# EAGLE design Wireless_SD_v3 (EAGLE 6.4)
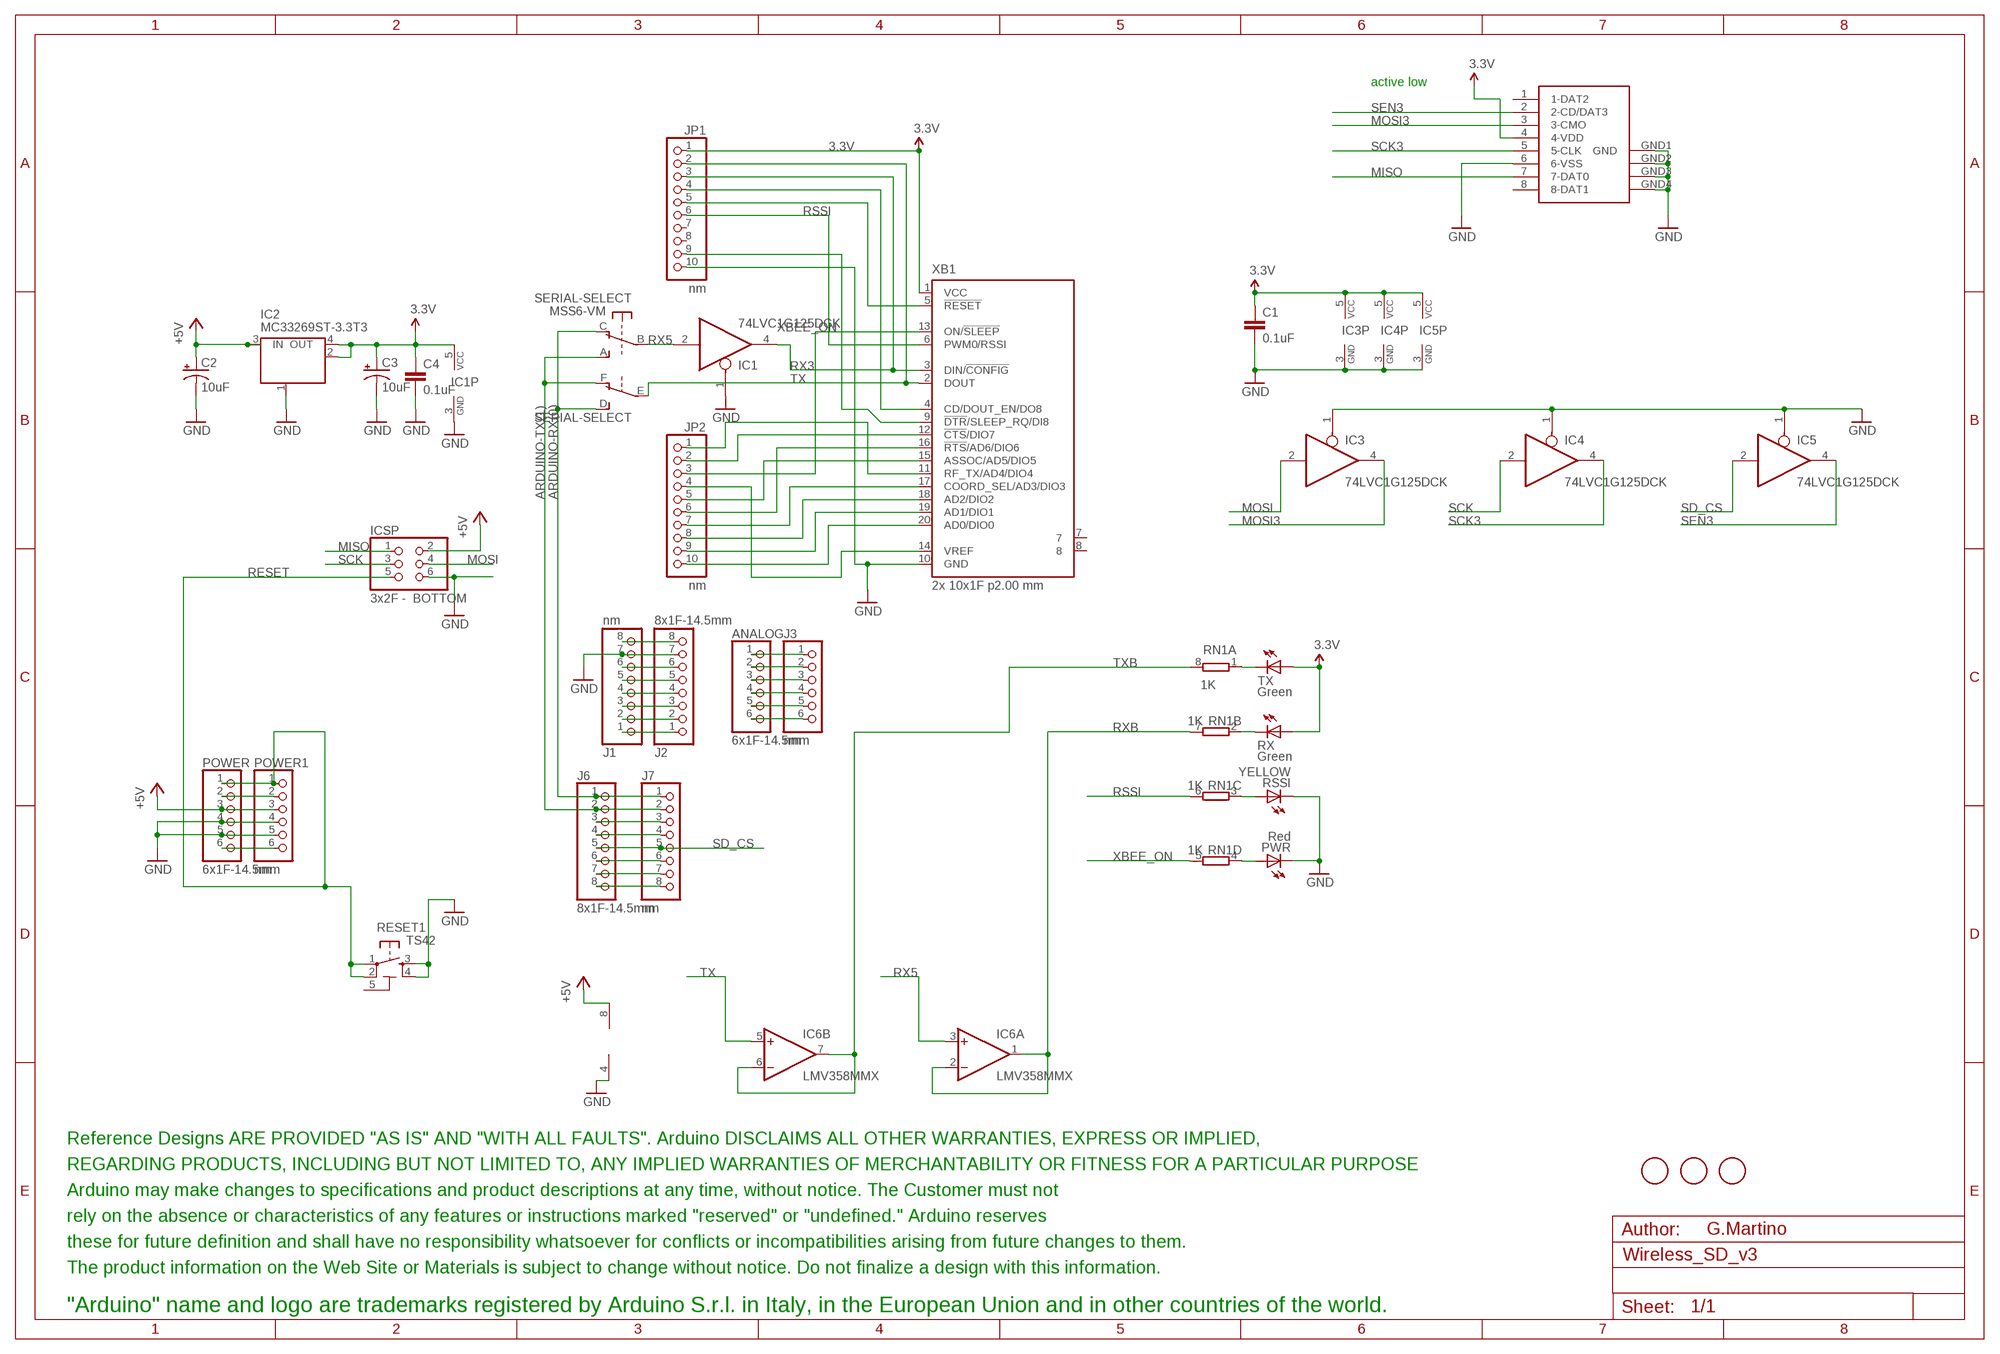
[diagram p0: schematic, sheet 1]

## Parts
A1  FIDUCIALMOUNT  [FIDUCIA-MOUNT]
A2  FIDUCIALMOUNT  [FIDUCIA-MOUNT]
A3  FIDUCIALMOUNT  [FIDUCIA-MOUNT]
ANALOG  6x1F-14.5mm  PINHD-1X6  [1X06]
C1  0.1uF  CAP0603-CAP  [0603-CAP]
C2  10uF  CAP_POL1206  [EIA3216]
C3  10uF  CAP_POL1206  [EIA3216]
C4  0.1uF  CAP0603-CAP  [0603-CAP]
IC1  74LVC1G125DCK  [SC70-5]
IC2  MC33269ST-3.3T3  [SOT223]
IC3  74LVC1G125DCK  [SC70-5]
IC4  74LVC1G125DCK  [SC70-5]
IC5  74LVC1G125DCK  [SC70-5]
IC6  LMV358MMX  [MSOP08]
ICSP  3x2F - BOTTOM  PINHD-2X3  [2X03]
J1  nm  PINHD-1X8  [1X08]
J2  8x1F-14.5mm  PINHD-1X8  [1X08]
J3  nm  PINHD-1X6  [1X06]
J6  8x1F-14.5mm  PINHD-1X8  [1X08]
J7  nm  PINHD-1X8  [1X08]
JP1  nm  PINHD-1X10  [1X10]
JP2  nm  PINHD-1X10  [1X10]
POWER  6x1F-14.5mm  PINHD-1X6  [1X06]
POWER1  nm  PINHD-1X6  [1X06]
PWR  Red  LEDCHIP-LED0805  [CHIP-LED0805]
RESET1  TS42  [TS42]
RN1  1K  4R-NCAY16  [CAY16]
RSSI  YELLOW  LEDCHIP-LED0805  [CHIP-LED0805]
RX  Green  LEDCHIP-LED0805  [CHIP-LED0805]
SERIAL-SELECT  MSS6-VM  [MSS6-V]
TX  Green  LEDCHIP-LED0805  [CHIP-LED0805]
U$2  DISCLAIMER-SMALL  [DISCLAIMER]
X1  SDCARD-15TW-8821  [SDCARD-15TW-8821]
XB1  2x 10x1F p2.00 mm  XBEE-PRO  [XBEE-PRO]

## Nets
3.3V: C1.1 C3.A(+) C4.1 IC1.5(VCC) IC2.2(OUT) IC2.4(OUT) IC3.5(VCC) IC4.5(VCC) IC5.5(VCC) JP1.1 RX.A TX.A X1.4(4-VDD) XB1.1(VCC)
+5V: C2.A(+) IC2.3(IN) IC6.8(P:V+) ICSP.2 POWER1.3 POWER.3
ARDUINO-RX(0): J6.1 J7.1 SERIAL-SELECT.C(O) SERIAL-SELECT.D(S)
ARDUINO-TX(1): J6.2 J7.2 SERIAL-SELECT.A(S) SERIAL-SELECT.F(O)
GND: C1.2 C2.C(-) C3.C(-) C4.2 IC1.1(OE) IC1.3(GND) IC2.1(GND/ADJ) IC3.1(OE) IC3.3(GND) IC4.1(OE) IC4.3(GND) IC5.1(OE) IC5.3(GND) IC6.4(P:V-) ICSP.6 J1.7 J2.7 JP1.10 POWER1.4 POWER1.5 POWER.4 POWER.5 PWR.C RESET1.3 RESET1.4 RSSI.C X1.6(6-VSS) X1.GND1(GND) X1.GND2(GND1) X1.GND3(GND2) X1.GND4(GND3) XB1.10(GND)
MISO: ICSP.1 X1.7(7-DAT0)
MOSI: IC3.2(I) ICSP.4
MOSI3: IC3.4(O) X1.3(3-CMO)
N$1: RN1.1 TX.C
N$2: J1.1 J2.1
N$5: RN1.2 RX.C
N$6: J1.2 J2.2
N$7: J1.3 J2.3
N$9: J1.6 J2.6
N$10: J6.3 J7.3
N$11: J6.4 J7.4
N$13: J6.6 J7.6
N$14: J6.7 J7.7
N$15: J6.8 J7.8
N$16: RN1.3 RSSI.A
N$18: ANALOG.1 J3.1
N$19: ANALOG.2 J3.2
N$20: ANALOG.3 J3.3
N$21: ANALOG.4 J3.4
N$22: ANALOG.5 J3.5
N$23: ANALOG.6 J3.6
N$24: JP2.10 XB1.20(AD0/DIO0)
N$25: JP2.9 XB1.19(AD1/DIO1)
N$27: J1.5 J2.5
N$28: JP2.8 XB1.18(AD2/DIO2)
N$29: PWR.A RN1.4
N$30: POWER1.6 POWER.6
N$33: JP2.7 XB1.17(COORD_SEL/AD3/DIO3)
N$34: JP2.6 XB1.16(!RTS!/AD6/DIO6)
N$36: JP2.5 XB1.15(ASSOC/AD5/DIO5)
N$37: JP2.4 XB1.14(VREF)
N$39: JP2.2 XB1.12(!CTS!/DIO7)
N$41: JP2.1 XB1.11(RF_TX/AD4/DIO4)
N$43: JP1.4 XB1.4(CD/DOUT_EN/DO8)
N$48: JP1.5 XB1.5(!RESET)
N$50: JP1.9 XB1.9(!DTR!/SLEEP_RQ/DI8)
N$61: J1.4 J2.4
N$222: J1.8 J2.8
N$223: POWER1.2 POWER.2
RESET: ICSP.5 POWER1.1 POWER.1 RESET1.1 RESET1.2
RSSI: JP1.6 RN1.6 XB1.6(PWM0/RSSI)
RX3: IC1.4(O) JP1.3 XB1.3(DIN/!CONFIG)
RX5: IC1.2(I) IC6.3(A:+IN) SERIAL-SELECT.B(P)
RXB: IC6.1(A:OUT) IC6.2(A:-IN) RN1.7
SCK: IC4.2(I) ICSP.3
SCK3: IC4.4(O) X1.5(5-CLK)
SD_CS: IC5.2(I) J6.5 J7.5
SEN3: IC5.4(O) X1.2(2-CD/DAT3)
TX: IC6.5(B:+IN) JP1.2 SERIAL-SELECT.E(P) XB1.2(DOUT)
TXB: IC6.6(B:-IN) IC6.7(B:OUT) RN1.8
XBEE_ON: JP2.3 RN1.5 XB1.13(ON/!SLEEP)
Unconnected: JP1.7 JP1.8 X1.1(1-DAT2) X1.8(8-DAT1) XB1.7 XB1.8

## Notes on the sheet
- active low
- G.Martino

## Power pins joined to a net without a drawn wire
5-GND: RESET1.5(5-GND)

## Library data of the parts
A1-A3 = Smartprj:FIDUCIALMOUNT
ANALOG J3 POWER POWER1 = pinhead:PINHD-1X6: PIN HEADER
C1 C4 = SparkFun:CAP: Capacitor
C2 C3 = SparkFun:CAP_POL: Capacitor Polarized
IC1 IC3-IC5 = 74xx-little-us:74*1G125: Single Bus Buffer Gate with 3-State Output
IC2 = linear:MC33269ST*: Adjustable Output Low Dropout Voltage Regulator 800 mA Source: http://www.onsemi.com/pub/Collateral/MC33269-D.PDF
IC6 = linear:LMV358?*: Dual General Purpose, Low Voltage, Rail-to-Rail Output Operational Amplifiers Source: http://www.national.com/mpf/LM/LMV321.html http://www.national.com/dt/lmv_qual.pdf
ICSP = pinhead:PINHD-2X3: PIN HEADER
J1 J2 J6 J7 = pinhead:PINHD-1X8: PIN HEADER
JP1 JP2 = pinhead:PINHD-1X10: PIN HEADER
PWR RSSI RX TX = led:LED: LED
RESET1 = st-mod v1.4:TS42: TS42 Dongnan Electronics Tact switch VDC 12V - 50mA
RN1 = resistor-dil:4R-N: Array Chip Resistor Source: RS Component / Phycomp
SERIAL-SELECT = Smartprj:MSS6-V
U$2 = Misc:DISCLAIMER-SMALL: DISCLAIMER
X1 = st-mod v1.3:SDCARD-15TW-8821: SD Card SDCARD 15TW 8821
XB1 = maxstream:XBEE: XBee (TM) /XBee-PRO(TM) OEM RF Modules Source: MaxStream, Inc. xbee_productmanual.pdf

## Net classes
0 default: width 0.203 mm, drill 0.559 mm, clearance 0.203 mm
1 power: width 0.152 mm, drill 0.61 mm, clearance 0.152 mm
2 gnd: width 0.203 mm, drill 0.559 mm, clearance 0.203 mm

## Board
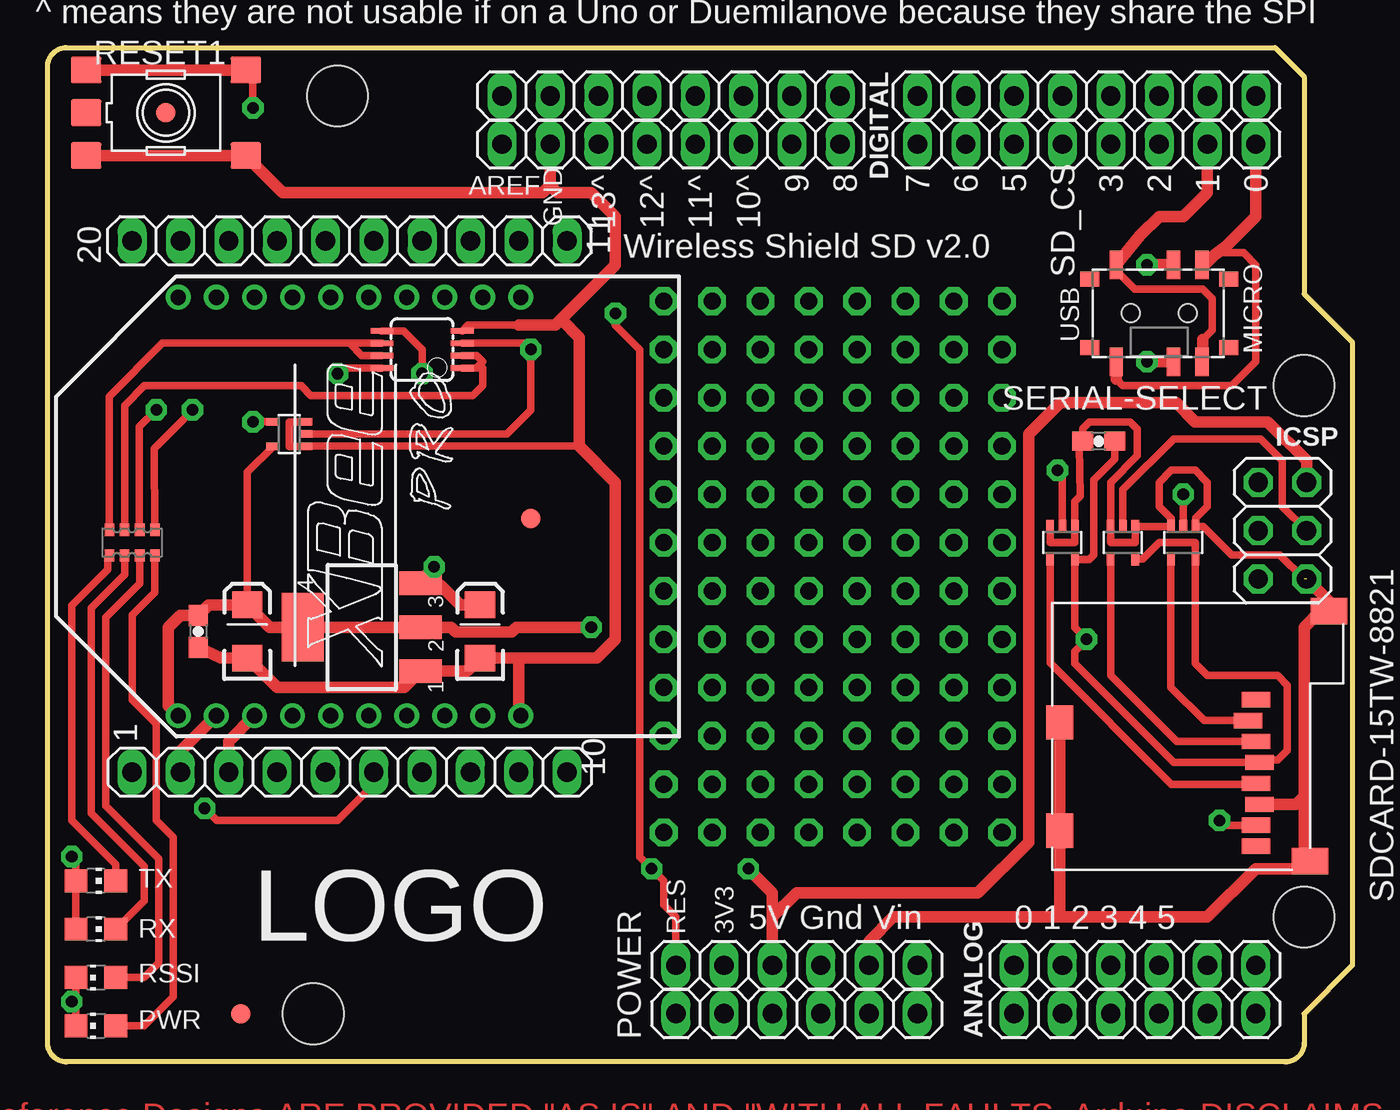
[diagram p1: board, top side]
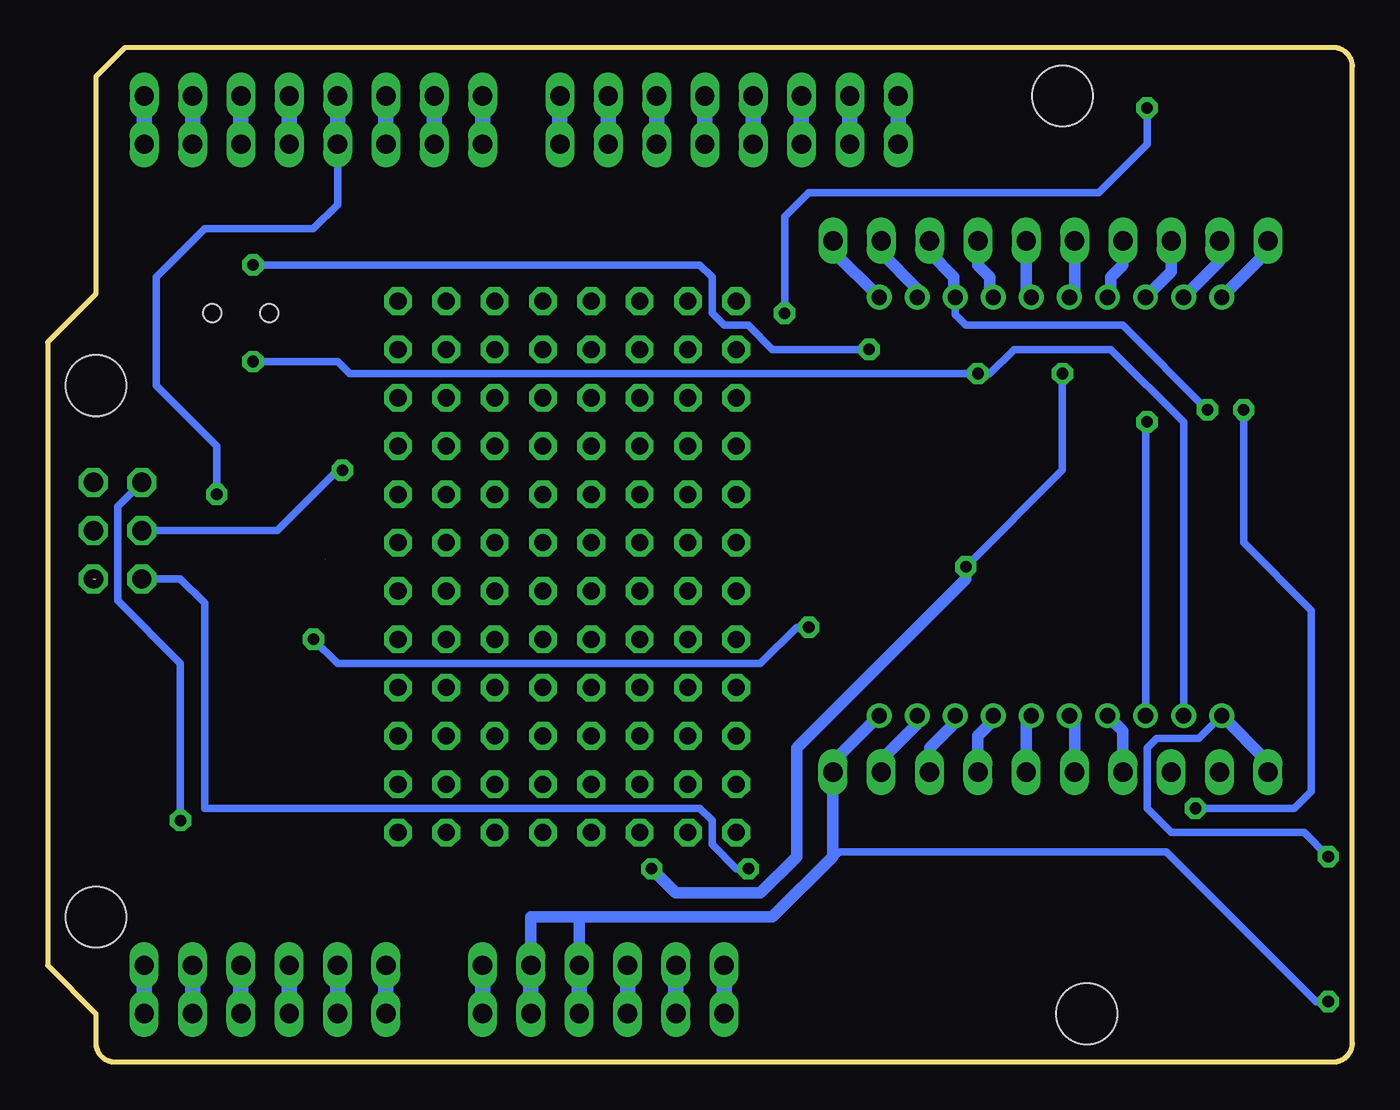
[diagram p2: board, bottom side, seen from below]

Size 68.58 x 53.34 mm. Coordinates in mm from the lower left corner, seen from the top.
Outline: 64.52,53.34 66.04,51.82 66.04,40.39 68.58,37.85 68.58,5.08 66.04,2.54 66.04,1 arc-90 65.04,0 1,0 arc-90 0,1 0,52.34 arc-90 1,53.34 64.52,53.34
Copper layers (1*16): Top 0.035mm / dielectric 1.5mm / Bottom 0.035mm
Design rules "ArduinoUno *": minimum track width 12mil, minimum drill 32mil, track to track 12mil, track to pad 12mil, pad to pad 12mil, via to via 12mil, smd to smd 12mil, copper to edge 32mil, drill to drill 16mil, minimum pad ring 10mil, minimum via ring 10mil, stop-mask expansion 2mil, vias tented up to drill 30mil, thermal gap 10mil
Holes 3.2 mm at 15.24,50.8 66.04,7.62 66.04,35.56 13.97,2.54

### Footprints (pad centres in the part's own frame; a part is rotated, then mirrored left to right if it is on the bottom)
FIDUCIA-MOUNT = smd 1.016 x 1.016: P$1 0,0
1X06 = drill 1.016 long: 1 -6.35,0; 2 -3.81,0; 3 -1.27,0; 4 1.27,0; 5 3.81,0; 6 6.35,0
0603-CAP = smd 1.1 x 1: 1 -0.85,0; 2 0.85,0
EIA3216 = smd 1.4 x 1.6: A 1.4,0; C -1.4,0
SC70-5 = smd 0.4 x 0.7: 1 -0.65,-0.85; 2 0,-0.85; 3 0.65,-0.85; 4 0.65,0.85; 5 -0.65,0.85
SOT223 = smd 1.219 x 2.235: 1 -2.311,-3.099; 2 0,-3.099; 3 2.311,-3.099 | smd 3.6 x 2.2: 4 0,3.099
MSOP08 = smd 0.3 x 1.2: 1 -0.976,-2.113; 2 -0.326,-2.113; 3 0.324,-2.113; 4 0.974,-2.113; 5 0.974,2.112; 6 0.324,2.112; 7 -0.326,2.112; 8 -0.976,2.112
2X03 = drill 1.016 octagon: 1 -2.54,-1.27; 2 -2.54,1.27; 3 0,-1.27; 4 0,1.27; 5 2.54,-1.27; 6 2.54,1.27
1X08 = drill 1.016 long: 1 -8.89,0; 2 -6.35,0; 3 -3.81,0; 4 -1.27,0; 5 1.27,0; 6 3.81,0; 7 6.35,0; 8 8.89,0
1X10 = drill 1.016 long: 1 -11.43,0; 2 -8.89,0; 3 -6.35,0; 4 -3.81,0; 5 -1.27,0; 6 1.27,0; 7 3.81,0; 8 6.35,0; 9 8.89,0; 10 11.43,0
CHIP-LED0805 = smd 1.2 x 1.2: A 0,-1.05; C 0,1.05
TS42 = smd 1.6 x 1.4: 1 -4.2,2.25; 2 4.2,2.25; 3 -4.2,-2.25; 4 4.2,-2.25; 5 -4.2,0
CAY16 = smd 0.5 x 0.65: 1 -1.2,-0.675; 2 -0.4,-0.675; 3 0.4,-0.675; 4 1.2,-0.675; 5 1.2,0.675; 6 0.4,0.675; 7 -0.4,0.675; 8 -1.2,0.675
MSS6-V = smd 1 x 0.8: 7 -3.65,1.8; 8 -3.65,-1.8; 9 3.65,1.8; 10 3.65,-1.8 | smd 0.7 x 1.5: A -2.25,2.55; B 0.75,2.55; C 2.25,2.55; D -2.25,-2.55; E 0.75,-2.55; F 2.25,-2.55 | hole 0.95: -1.5,0; 1.5,0
SDCARD-15TW-8821 = smd 0.8 x 1.5: 1 0,0; 2 1.1,-0.4; 3 2.2,0; 4 3.3,0.2; 5 4.4,0; 6 5.5,0.2; 7 6.6,0; 8 7.7,0 | smd 1.4 x 1.9: GND1 -4.66,3.85; GND2 8.49,2.85 | smd 1.8 x 1.4: GND3 1.19,-10.3; GND4 6.89,-10.3
XBEE-PRO = drill 0.8 pad 1.27: 1 -11,9; 2 -11,7; 3 -11,5; 4 -11,3; 5 -11,1; 6 -11,-1; 7 -11,-3; 8 -11,-5; 9 -11,-7; 10 -11,-9; 11 11,-9; 12 11,-7; 13 11,-5; 14 11,-3; 15 11,-1; 16 11,1; 17 11,3; 18 11,5; 19 11,7; 20 11,9

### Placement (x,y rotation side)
A1  10.16,2.54 0 top
A2  6.22,49.91 0 top
A3  25.4,28.57 0 top
ANALOG  57.15,2.54 0 top
C1  55.24,32.64 180 top
C2  22.73,22.64 90 top
C3  10.49,22.64 90 top
C4  7.92,22.64 270 top
IC1  12.7,33.02 90 top
IC2  16.51,22.86 90 top
IC3  56.52,27.3 180 top
IC4  53.34,27.3 180 top
IC5  59.69,27.3 180 top
IC6  19.68,37.47 90 top
ICSP  64.9,27.94 270 top
J1  32.77,48.26 180 top
J2  32.77,50.8 180 top
J3  57.15,5.08 0 top
J6  54.61,50.8 180 top
J7  54.61,48.26 180 top
JP1  15.88,15.24 0 top
JP2  15.88,43.18 180 top
POWER  39.37,2.54 0 top
POWER1  39.37,5.08 0 top
PWR  2.54,1.91 90 top
RESET1  6.22,49.91 0 top
RN1  4.45,27.3 0 top
RSSI  2.54,4.45 90 top
RX  2.54,6.99 270 top
SERIAL-SELECT  58.42,39.37 0 top
TX  2.54,9.53 270 top
U$2  not placed on the board
X1  63.5,19.05 270 top
XB1  15.88,29.21 90 top

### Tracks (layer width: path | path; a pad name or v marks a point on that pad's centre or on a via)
3.3V  (via drill 0.61)  (1 unrouted)
  Top 0.406: C1.1 56.09,31.71 54.99,30.61 54.99,26.67 54.74,26.42 54.03,26.42 IC4.5 | C3.A 10.49,31.02 IC1.5 | 60.33,26.47 60.33,20.95 60.96,20.32 64.64,20.32 65.15,19.81 65.15,16.38 64.64,15.88 63.83,15.88 X1.4 59.18,15.75 53.98,20.95 53.98,21.59 v54.61,22.23 53.98,22.86 53.98,26.44 | RX.A TX.A 1.49,10.57 v1.27,10.79 | IC3.5 57.57,26.45 58.42,27.3 60.33,27.3 60.33,26.47 | 60.33,26.47 IC5.5
  Top 0.61: v28.57,22.86 24.64,22.86 24.38,22.61 21.46,22.61 21.21,22.86 IC2.2 IC2.4 11.67,22.86 C3.A 8.46,24.04 C4.1 6.97,23.48 6.35,22.86 6.35,18.72 6.37,18.72 XB1.1
  Bottom 0.406: v1.27,10.79 2.54,12.06 9.53,12.06 10.79,13.34 10.79,16.51 10.29,17.02 8.07,17.02 XB1.1 | v28.57,22.86 29.21,22.86 31.11,20.95 53.34,20.95 v54.61,22.23
  Bottom 0.61: JP1.1 4.45,15.78 XB1.1
+5V  (via drill 0.61)
  Top 0.406: IC6.8 15.53,36.49 v15.24,36.2
  Top 0.61: 38.1,7.62 POWER1.3 | 38.1,7.62 39.37,8.89 48.9,8.89 51.56,11.56 51.56,33.02 53.21,34.67 59.31,34.67 60.33,33.66 64.14,33.66 66.17,31.62 ICSP.2 | 38.1,7.62 38.1,8.89 v36.83,10.16 | v20.32,26.04 19.61,25.32 IC2.3 19.7,25.08 20.64,25.08 21.68,24.04 C2.A
  Bottom 0.406: v15.24,36.2 15.24,31.11 v20.32,26.04
  Bottom 0.61: v36.83,10.16 35.56,8.89 31.11,8.89 29.21,10.79 29.21,16.51 20.32,25.4 v20.32,26.04
  Bottom 0.813: POWER1.3 POWER.3
ARDUINO-RX(0)
  Top 0.406: SERIAL-SELECT.C 60.97,41.92 61.59,42.55 62.87,42.55 63.5,41.91 63.5,36.83 62.23,35.56 56.52,35.56 56.17,35.91
  Top 0.61: SERIAL-SELECT.C 61.94,42.89 63.5,44.45 J7.1 | SERIAL-SELECT.D 56.17,35.91
  Bottom 0.813: J7.1 J6.1
ARDUINO-TX(1)
  Top 0.406: SERIAL-SELECT.A 56.17,41.62 57.15,40.64 60.71,40.64 61.21,40.13 61.21,38.48 60.71,37.97 | SERIAL-SELECT.F 60.71,36.86
  Top 0.61: SERIAL-SELECT.A 57.44,43.47 58.42,44.45 59.69,44.45 60.96,45.72 J7.2 | 60.71,36.86 60.71,37.97
  Bottom 0.813: J7.2 J6.2
GND  (via drill 0.61)  (1 unrouted)
  Top 0.406: PWR.C RSSI.C 1.49,3.4 v1.27,3.17 | 66.04,25.4 64.77,26.67 62.23,26.67 60.74,28.16 IC5.1 60.34,28.59 60.96,29.21 60.96,30.48 60.33,31.11 59.05,31.11 58.42,30.48 58.42,29.21 59.05,28.57 59.05,28.17 IC5.3 IC3.1 57.16,27.32 57.15,27.3 55.88,27.3 55.88,28.14 IC3.3 55.87,30.46 57.28,31.88 57.28,33.27 56.9,33.66 54.74,33.66 54.4,33.31 C1.2 54.23,32.47 54.23,32.38 54.27,29.76 53.99,29.48 IC4.1 53.98,28.14 53.98,27.3 52.7,27.3 52.69,27.32 IC4.3 | 24.77,38.73 22.09,38.73 IC6.4 | IC1.3 13.54,33.66 12.7,33.66 12.7,32.38 12.71,32.37 IC1.1 13.56,32.38 27.94,32.38
  Top 0.61: RESET1.3 RESET1.4 12.36,45.72 26.04,45.72 26.42,46.1 | C4.2 9.1,21.23 C3.C 10.52,21.23 12.06,19.68 18.75,19.68 IC2.1 22.05,20.55 C2.C 24.77,21.23 | XB1.10 24.77,18.32 24.77,21.23 | 26.42,46.1 J1.7 | 24.77,38.73 26.67,38.73 26.99,39.05 | 26.99,39.05 29.84,41.91 29.84,44.45 28.57,45.72 26.8,45.72 26.42,46.1 | 26.99,39.05 27.94,38.1 27.94,32.38 29.84,30.48 29.84,22.23 28.86,21.23 24.77,21.23 | POWER1.5 43.18,6.35 44.45,7.62 53.34,7.62 | 53.34,7.62 60.96,7.62 63.5,10.16 65.95,10.16 X1.GND2 66.04,10.87 66.04,13.97 | 66.04,13.97 66.04,22.86 66.89,23.71 X1.GND1 67.35,24.22 ICSP.6 | X1.6 65.62,13.55 66.04,13.97 | X1.GND4 X1.GND3 | X1.GND4 53.2,11.57 53.34,11.43 53.34,12.02 X1.GND4 | X1.GND4 53.2,7.76 53.34,7.62
  Bottom 0.406: v1.27,3.17 1.91,3.17 9.78,11.05 26.92,11.05 27.3,10.79
  Bottom 0.61: XB1.10 27.3,15.78 JP1.10 27.3,10.79 30.48,7.62 40.64,7.62 | 40.64,7.62 POWER1.4 | POWER1.5 43.18,7.62 40.64,7.62
  Bottom 0.813: J1.7 J2.7 | POWER1.4 POWER.4 | POWER1.5 POWER.5
MISO  (via drill 0.61)
  Top 0.406: X1.7 61.84,12.45 v61.59,12.7
  Bottom 0.406: v61.59,12.7 61.59,20.95 64.9,24.26 64.9,29.21 ICSP.1
MOSI
  Top 0.406: ICSP.4 64.9,29.21 64.9,31.62 63.75,32.77 59.18,32.77 56.52,30.1 IC3.2
MOSI3
  Top 0.406: IC3.4 55.87,20.34 59.35,16.85 X1.3
N$1
  Top 0.406: TX.C 3.59,10.38 1.27,12.7 1.27,24 3.17,25.91 3.17,26.56 RN1.1
N$2
  Bottom 0.813: J1.1 J2.1
N$5
  Top 0.406: RN1.2 4.04,25.64 2.29,23.88 2.29,13.08 5.08,10.29 5.08,8.47 RX.C
N$6
  Bottom 0.813: J1.2 J2.2
N$7
  Bottom 0.813: J1.3 J2.3
N$8  (via drill 0.9 pad 1.45)
  other vias: 34.92,32.38
N$9
  Bottom 0.813: J1.6 J2.6
N$10
  Bottom 0.813: J7.3 J6.3
N$11
  Bottom 0.813: J7.4 J6.4
N$13
  Bottom 0.813: J7.6 J6.6
N$14
  Bottom 0.813: J7.7 J6.7
N$15
  Bottom 0.813: J7.8 J6.8
N$16
  Top 0.406: RSSI.A 5.08,4.45 5.84,5.21 5.84,10.67 3.05,13.46 3.05,23.37 4.84,25.16 RN1.3
N$18
  Bottom 0.813: ANALOG.1 J3.1
N$19
  Bottom 0.813: ANALOG.2 J3.2
N$20
  Bottom 0.813: ANALOG.3 J3.3
N$21
  Bottom 0.813: ANALOG.4 J3.4
N$22
  Bottom 0.813: ANALOG.5 J3.5
N$23
  Bottom 0.813: ANALOG.6 J3.6
N$24
  Bottom 0.61: JP2.10 4.45,42.64 XB1.20
N$25
  Bottom 0.61: JP2.9 6.99,42.1 XB1.19
N$27
  Bottom 0.813: J1.5 J2.5
N$28
  Bottom 0.61: JP2.8 9.53,41.56 XB1.18
N$29
  Top 0.406: PWR.A 5.08,1.91 6.6,3.43 6.6,11.81 5.71,12.7 5.71,17.78 4.45,19.05 4.45,23.5 5.64,24.7 RN1.4
N$30
  Bottom 0.813: POWER.6 POWER1.6
N$32  (via drill 0.9 pad 1.45)
  other vias: 34.92,40.01
N$33
  Bottom 0.61: JP2.7 12.06,41.91 12.7,41.27 12.7,40.38 XB1.17
N$34
  Bottom 0.61: JP2.6 14.61,40.48 XB1.16
N$35  (via drill 0.9 pad 1.45)
  other vias: 34.92,37.47
N$36
  Bottom 0.61: JP2.5 17.14,40.48 XB1.15
N$37
  Bottom 0.61: JP2.4 19.68,41.91 19.05,41.27 19.05,40.38 XB1.14
N$38  (via drill 0.9 pad 1.45)
  other vias: 34.92,34.92
N$39
  Bottom 0.61: JP2.2 24.77,42.55 22.86,40.64 22.86,40.23 XB1.12
N$41
  Bottom 0.61: JP2.1 27.3,42.64 XB1.11
N$43
  Bottom 0.61: JP1.4 12.06,17.4 XB1.4
N$48
  Bottom 0.61: JP1.5 14.61,17.94 XB1.5
N$50
  Bottom 0.61: JP1.9 24.77,15.88 22.86,17.78 22.86,18.2 XB1.9
N$55  (via drill 0.9 pad 1.45)
  other vias: 34.92,29.84
N$57  (via drill 0.9 pad 1.45)
  other vias: 34.92,27.3
N$58  (via drill 0.9 pad 1.45)
  other vias: 34.92,24.77
N$60  (via drill 0.9 pad 1.45)
  other vias: 50.16,40.01
N$61
  Bottom 0.813: J1.4 J2.4
N$62  (via drill 0.9 pad 1.45)
  other vias: 45.09,40.01
N$63  (via drill 0.9 pad 1.45)
  other vias: 34.92,22.23
N$64  (via drill 0.9 pad 1.45)
  other vias: 40.01,40.01
N$65  (via drill 0.9 pad 1.45)
  other vias: 34.92,19.68
N$66  (via drill 0.9 pad 1.45)
  other vias: 34.92,17.14
N$67  (via drill 0.9 pad 1.45)
  other vias: 34.92,14.61
N$68  (via drill 0.9 pad 1.45)
  other vias: 34.92,12.06
N$69  (via drill 0.9 pad 1.45)
  other vias: 32.38,32.38
N$70  (via drill 0.9 pad 1.45)
  other vias: 32.38,29.84
N$71  (via drill 0.9 pad 1.45)
  other vias: 32.38,27.3
N$72  (via drill 0.9 pad 1.45)
  other vias: 32.38,24.77
N$75  (via drill 0.9 pad 1.45)
  other vias: 32.38,22.23
N$76  (via drill 0.9 pad 1.45)
  other vias: 42.55,40.01
N$77  (via drill 0.9 pad 1.45)
  other vias: 37.47,40.01
N$79  (via drill 0.9 pad 1.45)
  other vias: 50.16,37.47
N$80  (via drill 0.9 pad 1.45)
  other vias: 45.09,37.47
N$81  (via drill 0.9 pad 1.45)
  other vias: 40.01,37.47
N$82  (via drill 0.9 pad 1.45)
  other vias: 32.38,19.68
N$85  (via drill 0.9 pad 1.45)
  other vias: 47.62,40.01
N$86  (via drill 0.9 pad 1.45)
  other vias: 42.55,37.47
N$87  (via drill 0.9 pad 1.45)
  other vias: 37.47,37.47
N$89  (via drill 0.9 pad 1.45)
  other vias: 50.16,34.92
N$90  (via drill 0.9 pad 1.45)
  other vias: 45.09,34.92
N$91  (via drill 0.9 pad 1.45)
  other vias: 40.01,34.92
N$92  (via drill 0.9 pad 1.45)
  other vias: 32.38,17.14
N$95  (via drill 0.9 pad 1.45)
  other vias: 47.62,34.92
N$96  (via drill 0.9 pad 1.45)
  other vias: 42.55,34.92
N$97  (via drill 0.9 pad 1.45)
  other vias: 37.47,34.92
N$99  (via drill 0.9 pad 1.45)
  other vias: 50.16,32.38
N$100  (via drill 0.9 pad 1.45)
  other vias: 45.09,32.38
N$101  (via drill 0.9 pad 1.45)
  other vias: 40.01,32.38
N$102  (via drill 0.9 pad 1.45)
  other vias: 32.38,14.61
N$105  (via drill 0.9 pad 1.45)
  other vias: 47.62,32.38
N$106  (via drill 0.9 pad 1.45)
  other vias: 42.55,32.38
N$107  (via drill 0.9 pad 1.45)
  other vias: 37.47,32.38
N$109  (via drill 0.9 pad 1.45)
  other vias: 50.16,29.84
N$110  (via drill 0.9 pad 1.45)
  other vias: 45.09,29.84
N$111  (via drill 0.9 pad 1.45)
  other vias: 40.01,29.84
N$112  (via drill 0.9 pad 1.45)
  other vias: 32.38,12.06
N$115  (via drill 0.9 pad 1.45)
  other vias: 47.62,29.84
N$116  (via drill 0.9 pad 1.45)
  other vias: 42.55,29.84
N$117  (via drill 0.9 pad 1.45)
  other vias: 37.47,29.84
N$119  (via drill 0.9 pad 1.45)
  other vias: 50.16,27.3
N$120  (via drill 0.9 pad 1.45)
  other vias: 45.09,27.3
N$121  (via drill 0.9 pad 1.45)
  other vias: 40.01,27.3
N$122  (via drill 0.9 pad 1.45)
  other vias: 32.38,40.01
N$125  (via drill 0.9 pad 1.45)
  other vias: 47.62,27.3
N$126  (via drill 0.9 pad 1.45)
  other vias: 42.55,27.3
N$127  (via drill 0.9 pad 1.45)
  other vias: 37.47,27.3
N$129  (via drill 0.9 pad 1.45)
  other vias: 50.16,24.77
N$130  (via drill 0.9 pad 1.45)
  other vias: 45.09,24.77
N$131  (via drill 0.9 pad 1.45)
  other vias: 40.01,24.77
N$132  (via drill 0.9 pad 1.45)
  other vias: 32.38,37.47
N$135  (via drill 0.9 pad 1.45)
  other vias: 47.62,24.77
N$136  (via drill 0.9 pad 1.45)
  other vias: 42.55,24.77
N$137  (via drill 0.9 pad 1.45)
  other vias: 37.47,24.77
N$139  (via drill 0.9 pad 1.45)
  other vias: 50.16,22.23
N$140  (via drill 0.9 pad 1.45)
  other vias: 45.09,22.23
N$141  (via drill 0.9 pad 1.45)
  other vias: 40.01,22.23
N$142  (via drill 0.9 pad 1.45)
  other vias: 32.38,34.92
N$145  (via drill 0.9 pad 1.45)
  other vias: 47.62,22.23
N$146  (via drill 0.9 pad 1.45)
  other vias: 42.55,22.23
N$147  (via drill 0.9 pad 1.45)
  other vias: 37.47,22.23
N$149  (via drill 0.9 pad 1.45)
  other vias: 50.16,19.68
N$150  (via drill 0.9 pad 1.45)
  other vias: 45.09,19.68
N$151  (via drill 0.9 pad 1.45)
  other vias: 40.01,19.68
N$152  (via drill 0.9 pad 1.45)
  other vias: 47.62,37.47
N$155  (via drill 0.9 pad 1.45)
  other vias: 47.62,19.68
N$156  (via drill 0.9 pad 1.45)
  other vias: 42.55,19.68
N$157  (via drill 0.9 pad 1.45)
  other vias: 37.47,19.68
N$159  (via drill 0.9 pad 1.45)
  other vias: 50.16,17.14
N$160  (via drill 0.9 pad 1.45)
  other vias: 45.09,17.14
N$161  (via drill 0.9 pad 1.45)
  other vias: 40.01,17.14
N$165  (via drill 0.9 pad 1.45)
  other vias: 47.62,17.14
N$166  (via drill 0.9 pad 1.45)
  other vias: 42.55,17.14
N$167  (via drill 0.9 pad 1.45)
  other vias: 37.47,17.14
N$169  (via drill 0.9 pad 1.45)
  other vias: 50.16,14.61
N$170  (via drill 0.9 pad 1.45)
  other vias: 45.09,14.61
N$171  (via drill 0.9 pad 1.45)
  other vias: 40.01,14.61
N$175  (via drill 0.9 pad 1.45)
  other vias: 47.62,14.61
N$176  (via drill 0.9 pad 1.45)
  other vias: 42.55,14.61
N$177  (via drill 0.9 pad 1.45)
  other vias: 37.47,14.61
N$179  (via drill 0.9 pad 1.45)
  other vias: 50.16,12.06
N$180  (via drill 0.9 pad 1.45)
  other vias: 45.09,12.06
N$181  (via drill 0.9 pad 1.45)
  other vias: 40.01,12.06
N$185  (via drill 0.9 pad 1.45)
  other vias: 47.62,12.06
N$186  (via drill 0.9 pad 1.45)
  other vias: 42.55,12.06
N$187  (via drill 0.9 pad 1.45)
  other vias: 37.47,12.06
N$188
  Bottom 0.61: 18.92,18.16 18.92,17.91 19.68,17.14 19.68,15.88
N$190
  Bottom 0.61: 20.83,18.16 20.83,17.91 22.23,16.51 22.23,15.88
N$222
  Bottom 0.813: J1.8 J2.8
N$223
  Bottom 0.813: POWER.2 POWER1.2
RESET  (via drill 0.61)
  Top 0.406: POWER1.1 33.02,7.62 32.38,8.26 32.38,9.53 v31.75,10.16 31.11,10.79 31.11,37.47 29.84,38.73 v29.84,39.37 | RESET1.2 10.79,51.79 v10.79,50.16
  Top 0.61: RESET1.2 RESET1.1
  Bottom 0.406: ICSP.5 61.59,25.4 60.33,24.13 60.33,13.34 34.29,13.34 33.66,12.7 33.66,11.43 32.38,10.16 v31.75,10.16 | v10.79,50.16 10.79,48.26 13.34,45.72 28.57,45.72 29.84,44.45 v29.84,39.37
  Bottom 0.813: POWER.1 POWER1.1
RSSI  (via drill 0.61)
  Top 0.406: RN1.6 4.83,27.96 4.83,33.4 v5.71,34.29 | JP1.6 17.14,14.61 15.24,12.7 8.89,12.7 v8.26,13.34
  Bottom 0.406: v5.71,34.29 5.71,27.3 2.16,23.75 2.16,14.22 3.05,13.34 v8.26,13.34
  Bottom 0.61: JP1.6 17.14,17.94 XB1.6
RX3  (via drill 0.61)
  Top 0.406: IC1.4 10.81,33.67 v10.79,33.66
  Top 0.61: JP1.3 9.53,16.86 XB1.3
  Bottom 0.406: XB1.3 10.88,33.73 v10.79,33.66
RX5  (via drill 0.61)
  Top 0.406: v57.78,41.91 57.8,41.92 | IC6.3 25.08,37.79 v25.4,37.47 25.4,34.29 24.13,33.02 IC1.2
  Top 0.61: 57.8,41.92 SERIAL-SELECT.B
  Bottom 0.406: v57.78,41.91 34.29,41.91 33.66,41.27 33.66,39.37 33.02,38.73 31.75,38.73 30.48,37.47 28.57,37.47 v25.4,37.47
RXB
  Top 0.406: RN1.7 4.04,34.52 5.08,35.56 13.34,35.56 13.84,35.05 22.35,35.05 22.86,35.56 22.86,36.49 22.52,36.49 | IC6.2 22.55,37.14 22.86,36.83 22.52,36.49 | 22.52,36.49 IC6.1
SCK  (via drill 0.61)
  Top 0.406: IC4.2 53.34,30.48 53.34,30.86 v53.09,31.11
  Bottom 0.406: ICSP.3 56.52,27.94 53.34,31.11 v53.09,31.11
SCK3
  Top 0.406: IC4.4 52.69,20.97 59.05,14.61 63.45,14.61 X1.5
SD_CS  (via drill 0.61)
  Top 0.406: IC5.2 v59.69,29.84
  Bottom 0.406: J7.5 53.34,45.09 54.61,43.81 60.33,43.81 62.87,41.27 62.87,35.56 59.69,32.38 v59.69,29.84
  Bottom 0.813: J7.5 J6.5
SEN3
  Top 0.406: IC5.4 59.04,19.7 60.79,17.95 X1.2
TX  (via drill 0.61)
  Top 0.406: SERIAL-SELECT.E | IC6.5 18.71,38.44 19.68,37.47 v19.68,36.2
  Top 0.61: JP1.2 6.99,16.32 XB1.2 | v57.78,36.83 SERIAL-SELECT.E
  Bottom 0.406: v57.78,36.83 53.34,36.83 52.7,36.2 v19.68,36.2 19.05,36.2 17.78,37.47 12.7,37.47 8.88,33.64 XB1.2
TXB
  Top 0.406: RN1.8 3.25,34.99 6.04,37.79 15.88,37.79 | 15.88,37.79 IC6.6 | IC6.7 16.52,37.14 15.88,37.79
XBEE_ON  (via drill 0.61)
  Top 0.406: RN1.5 5.61,32.26 v7.62,34.29
  Bottom 0.406: v7.62,34.29 12.06,38.73 20.32,38.73 20.88,39.29 XB1.13
  Bottom 0.61: JP2.3 22.23,42.55 20.95,41.27 20.95,40.29 XB1.13

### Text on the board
tPlace: ^ means they are not usable if on a Uno or Duemilanove because they share the SPI | 9 | 8 | 7 | 6 | 5 | 3 | 2 | 1 | 0 | 13^ | 12^ | 11^ | 10^ | Wireless Shield SD v2.0 | SD_CS | LOGO
tNames: DIGITAL | AREF | GND | 20 | 11 | USB | MICRO | 1 | 10 | RES | 3V3 | 5V Gnd Vin | 0 1 2 3 4 5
